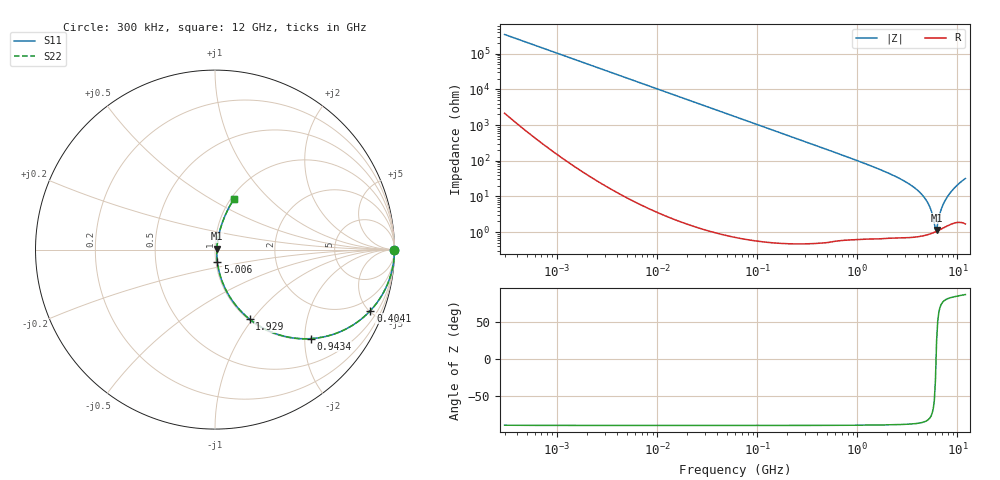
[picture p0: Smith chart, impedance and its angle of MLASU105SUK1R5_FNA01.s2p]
! MLASU105SUK1R5_FNA01  S-PARAMETER MODEL  ( General Type )
! Model Generated by TAIYO YUDEN Corporation (http://www.ty-top.com)
! Version 2.0
! TAIYO YUDEN Control No. 120810
! Copyright(c) 2011 TAIYO YUDEN CO.,LTD. All Rights Reserved.
! Product Description (link to TY-COMPAS)
! https://ds.yuden.co.jp/TYCOMPAS/or/detail?pn=MLASU105SUK1R5CFNA01&u=M
! Products Name : Multilayer Ceramic Capacitors
! Characteristics :
!  Capacitance : 1.5 pF , Rated Voltage : 50V , TCC : UK / U2K
!  Case Size : 1.0 x 0.5 / 0.039 x 0.02 [mm/inch] , Thickness : 0.5 / 0.02 [mm/inch]
!  (Conditions: Temperature = 25 degC , DC Bias Current/Voltage = 0A / 0V)
! External Node Assignments :
!  1  o---| |---o  2
! GND o---------o GND
! Frequency Range : 0.3MHz  -  12000MHz  [ 401 STEP ]
# MHz S RI R 50
! Freq[MHz].  S11 Real  S11 Imag  S21 Real  S21 Imag  S12 Real  S12 Imag  S22 Real  S22 Imag
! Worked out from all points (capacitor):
!   401 points, 300 kHz to 12 GHz, reference 50 ohm
!   read as one part in series: C = 1.54 pF near 316.3 kHz
!   lowest |Z| = 1.16 ohm at 6.188 GHz (marker M1)
!   series resonance near 6.114 GHz, so ESL is about 440 pH
!   S11 on the Smith chart (normalised r, x): 300 kHz: open; 404.1 MHz: 1.01, -5.10; 943.4 MHz: 1.01, -2.14; 1.929 GHz: 1.01, -0.97; 5.006 GHz: 1.02, -0.14; 12 GHz: 1.03, +0.64
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0.3  1 -0.00029  1.88e-06 0.00029  1.88e-06 0.00029  1 -0.00029
1.769972  1 -0.00171  4.41e-06 0.00171  4.41e-06 0.00171  1 -0.00171
10.44266  0.9999 -0.0101  0.000105 0.0101  0.000105 0.0101  0.9999 -0.0101
60  0.9966 -0.0578  0.00338 0.0578  0.00338 0.0578  0.9966 -0.0578
155.7172  0.9777 -0.1473  0.0223 0.1473  0.0223 0.1473  0.9777 -0.1473
353.9943  0.8941 -0.3069  0.1059 0.3069  0.1059 0.3069  0.8941 -0.3069
404.1309  0.8661 -0.3396  0.1339 0.3396  0.1339 0.3396  0.8661 -0.3396
601.3112  0.7431 -0.4353  0.2569 0.4353  0.2569 0.4353  0.7431 -0.4353
943.3804  0.5338 -0.496  0.4662 0.496  0.4662 0.496  0.5338 -0.496
1928.972  0.1927 -0.3876  0.8073 0.3876  0.8073 0.3876  0.1927 -0.3876
2088.533  0.1647 -0.3633  0.8353 0.3633  0.8353 0.3633  0.1647 -0.3633
3642.919  0.0392 -0.1755  0.9608 0.1755  0.9608 0.1755  0.0392 -0.1755
4385.161  0.0206 -0.1123  0.9794 0.1123  0.9794 0.1123  0.0206 -0.1123
5006.236  0.013 -0.0677  0.987 0.0677  0.987 0.0677  0.013 -0.0677
5420.343  0.0107 -0.0412  0.9893 0.0412  0.9893 0.0412  0.0107 -0.0412
5868.704  0.01 -0.0148  0.99 0.0148  0.99 0.0148  0.01 -0.0148
6188.031  0.0105 0.00464  0.9895 -0.00464  0.9895 -0.00464  0.0105 0.00464
6354.153  0.011 0.0134  0.989 -0.0134  0.989 -0.0134  0.011 0.0134
7064.448  0.0151 0.0501  0.9849 -0.0501  0.9849 -0.0501  0.0151 0.0501
7854.144  0.0228 0.0894  0.9772 -0.0894  0.9772 -0.0894  0.0228 0.0894
9708.23  0.0523 0.18  0.9477 -0.18  0.9477 -0.18  0.0523 0.18
12000  0.1046 0.2806  0.8954 -0.2806  0.8954 -0.2806  0.1046 0.2806
